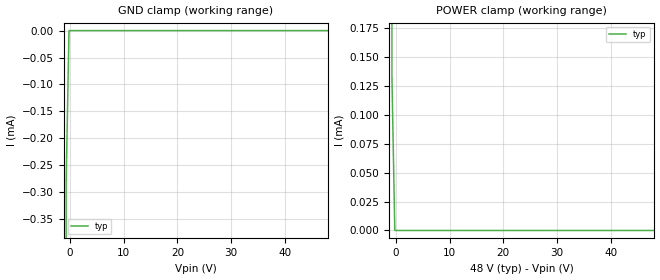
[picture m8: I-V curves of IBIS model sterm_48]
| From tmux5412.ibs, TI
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| sterm_48
[Model]   sterm_48
Model_type   Terminator
|   typ   min   max
C_comp   1.008417e-11   NA   NA
[Voltage Range]   48   NA   NA
[Temperature Range]   27   NA   NA
[Power Clamp Reference]   48   NA   NA
[GND Clamp Reference]   0   NA   NA
[GND Clamp]
|   Voltage   I(typ)   I(min)   I(max)
-5V       -2.839A    NA         NA
-1.253V   -90.92mA   NA         NA
-717.2mV  -285.5uA   NA         NA
-181.8mV  -1.964nA   NA         NA
48V       4.289nA    NA         NA
[POWER Clamp]
|   Voltage   I(typ)   I(min)   I(max)
-5V       2.611A     NA         NA
-1.252V   80.72mA    NA         NA
-717.2mV  133.1uA    NA         NA
-181.8mV  4.33nA     NA         NA
48V       -1.892nA   NA         NA
